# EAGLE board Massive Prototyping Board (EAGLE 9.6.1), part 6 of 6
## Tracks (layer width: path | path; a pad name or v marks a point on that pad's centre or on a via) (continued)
N$2069  (via drill 0.94) (continued)
  Bottom 2.032: v19.05,101.6 v21.59,101.6 v24.13,101.6 v26.67,101.6 v29.21,101.6
N$2070  (via drill 0.94)
  Bottom 2.032: v19.05,104.14 v21.59,104.14 v24.13,104.14 v26.67,104.14 v29.21,104.14
N$2071  (via drill 0.94)
  Bottom 2.032: v19.05,106.68 v21.59,106.68 v24.13,106.68 v26.67,106.68 v29.21,106.68
N$2072  (via drill 0.94)
  Bottom 2.032: v19.05,109.22 v21.59,109.22 v24.13,109.22 v26.67,109.22 v29.21,109.22
N$2073  (via drill 0.94)
  Bottom 2.032: v19.05,111.76 v21.59,111.76 v24.13,111.76 v26.67,111.76 v29.21,111.76
N$2074  (via drill 0.94)
  Bottom 2.032: v19.05,114.3 v21.59,114.3 v24.13,114.3 v26.67,114.3 v29.21,114.3
N$2075  (via drill 0.94)
  Bottom 2.032: v19.05,116.84 v21.59,116.84 v24.13,116.84 v26.67,116.84 v29.21,116.84
N$2076  (via drill 0.94)
  Bottom 2.032: v19.05,119.38 v21.59,119.38 v24.13,119.38 v26.67,119.38 v29.21,119.38
N$2077  (via drill 0.94)
  Bottom 2.032: v19.05,121.92 v21.59,121.92 v24.13,121.92 v26.67,121.92 v29.21,121.92
N$2078  (via drill 0.94)
  Bottom 2.032: v19.05,124.46 v21.59,124.46 v24.13,124.46 v26.67,124.46 v29.21,124.46
N$2079  (via drill 0.94)
  Bottom 2.032: v19.05,127 v21.59,127 v24.13,127 v26.67,127 v29.21,127
N$2080  (via drill 0.94)
  Bottom 2.032: v19.05,129.54 v21.59,129.54 v24.13,129.54 v26.67,129.54 v29.21,129.54
N$2081  (via drill 0.94)
  Bottom 2.032: v19.05,132.08 v21.59,132.08 v24.13,132.08 v26.67,132.08 v29.21,132.08
N$2082  (via drill 0.94)
  Bottom 2.032: v19.05,134.62 v21.59,134.62 v24.13,134.62 v26.67,134.62 v29.21,134.62
N$2083  (via drill 0.94)
  Bottom 2.032: v19.05,137.16 v21.59,137.16 v24.13,137.16 v26.67,137.16 v29.21,137.16
N$2084  (via drill 0.94)
  Bottom 2.032: v19.05,139.7 v21.59,139.7 v24.13,139.7 v26.67,139.7 v29.21,139.7
N$2085  (via drill 0.94)
  Bottom 2.032: v19.05,142.24 v21.59,142.24 v24.13,142.24 v26.67,142.24 v29.21,142.24
N$2086  (via drill 0.94)
  Bottom 2.032: v19.05,144.78 v21.59,144.78 v24.13,144.78 v26.67,144.78 v29.21,144.78
N$2087  (via drill 0.94)
  Bottom 2.032: v19.05,147.32 v21.59,147.32 v24.13,147.32 v26.67,147.32 v29.21,147.32
N$2088  (via drill 0.94)
  Bottom 2.032: v19.05,149.86 v21.59,149.86 v24.13,149.86 v26.67,149.86 v29.21,149.86
N$2089  (via drill 0.94)
  Bottom 2.032: v19.05,152.4 v21.59,152.4 v24.13,152.4 v26.67,152.4 v29.21,152.4
N$2090  (via drill 0.94)
  Bottom 2.032: v19.05,154.94 v21.59,154.94 v24.13,154.94 v26.67,154.94 v29.21,154.94
N$2091  (via drill 0.94)
  Bottom 2.032: v19.05,157.48 v21.59,157.48 v24.13,157.48 v26.67,157.48 v29.21,157.48
N$2092  (via drill 0.94)
  Bottom 2.032: v19.05,160.02 v21.59,160.02 v24.13,160.02 v26.67,160.02 v29.21,160.02
N$2093  (via drill 0.94)
  Bottom 2.032: v19.05,162.56 v21.59,162.56 v24.13,162.56 v26.67,162.56 v29.21,162.56
N$2094  (via drill 0.94)
  Bottom 2.032: v19.05,165.1 v21.59,165.1 v24.13,165.1 v26.67,165.1 v29.21,165.1
N$2095  (via drill 0.94)
  Bottom 2.032: v19.05,167.64 v21.59,167.64 v24.13,167.64 v26.67,167.64 v29.21,167.64
N$2096  (via drill 0.94)
  Bottom 2.032: v19.05,170.18 v21.59,170.18 v24.13,170.18 v26.67,170.18 v29.21,170.18
N$2097  (via drill 0.94)
  Bottom 2.032: v19.05,172.72 v21.59,172.72 v24.13,172.72 v26.67,172.72 v29.21,172.72
N$2098  (via drill 0.94)
  Bottom 2.032: v19.05,175.26 v21.59,175.26 v24.13,175.26 v26.67,175.26 v29.21,175.26
N$2099  (via drill 0.94)
  Bottom 2.032: v19.05,177.8 v21.59,177.8 v24.13,177.8 v26.67,177.8 v29.21,177.8
N$2100  (via drill 0.94)
  Bottom 2.032: v19.05,180.34 v21.59,180.34 v24.13,180.34 v26.67,180.34 v29.21,180.34
N$2101  (via drill 0.94)
  Bottom 2.032: v19.05,182.88 v21.59,182.88 v24.13,182.88 v26.67,182.88 v29.21,182.88
N$2102  (via drill 0.94)
  Bottom 2.032: v19.05,185.42 v21.59,185.42 v24.13,185.42 v26.67,185.42 v29.21,185.42
N$2103  (via drill 0.94)
  Bottom 2.032: v19.05,187.96 v21.59,187.96 v24.13,187.96 v26.67,187.96 v29.21,187.96
N$2104  (via drill 0.94)
  Bottom 2.032: v19.05,190.5 v21.59,190.5 v24.13,190.5 v26.67,190.5 v29.21,190.5
N$2105  (via drill 0.94)
  Bottom 2.032: v19.05,193.04 v21.59,193.04 v24.13,193.04 v26.67,193.04 v29.21,193.04
N$2106  (via drill 0.94)
  Bottom 2.032: v19.05,195.58 v21.59,195.58 v24.13,195.58 v26.67,195.58 v29.21,195.58
N$2107  (via drill 0.94)
  Bottom 2.032: v19.05,198.12 v21.59,198.12 v24.13,198.12 v26.67,198.12 v29.21,198.12
N$2108  (via drill 0.94)
  Bottom 2.032: v19.05,200.66 v21.59,200.66 v24.13,200.66 v26.67,200.66 v29.21,200.66
N$2109  (via drill 0.94)
  Bottom 2.032: v19.05,203.2 v21.59,203.2 v24.13,203.2 v26.67,203.2 v29.21,203.2
N$2110  (via drill 0.94)
  Bottom 2.032: v19.05,205.74 v21.59,205.74 v24.13,205.74 v26.67,205.74 v29.21,205.74
N$2111  (via drill 0.94)
  Bottom 2.032: v19.05,208.28 v21.59,208.28 v24.13,208.28 v26.67,208.28 v29.21,208.28
N$2112  (via drill 0.94)
  Bottom 2.032: v19.05,210.82 v21.59,210.82 v24.13,210.82 v26.67,210.82 v29.21,210.82
N$2113  (via drill 0.94)
  Bottom 2.032: v19.05,213.36 v21.59,213.36 v24.13,213.36 v26.67,213.36 v29.21,213.36
N$2114  (via drill 0.94)
  Bottom 2.032: v19.05,215.9 v21.59,215.9 v24.13,215.9 v26.67,215.9 v29.21,215.9
N$2115  (via drill 0.94)
  Bottom 2.032: v19.05,218.44 v21.59,218.44 v24.13,218.44 v26.67,218.44 v29.21,218.44
N$2116  (via drill 0.94)
  Bottom 2.032: v19.05,220.98 v21.59,220.98 v24.13,220.98 v26.67,220.98 v29.21,220.98
N$2117  (via drill 0.94)
  Bottom 2.032: v19.05,223.52 v21.59,223.52 v24.13,223.52 v26.67,223.52 v29.21,223.52
N$2118  (via drill 0.94)
  Bottom 2.032: v19.05,226.06 v21.59,226.06 v24.13,226.06 v26.67,226.06 v29.21,226.06
N$2119  (via drill 0.94)
  Bottom 2.032: v19.05,228.6 v21.59,228.6 v24.13,228.6 v26.67,228.6 v29.21,228.6
N$2120  (via drill 0.94)
  Bottom 2.032: v19.05,231.14 v21.59,231.14 v24.13,231.14 v26.67,231.14 v29.21,231.14
N$2121  (via drill 0.94)
  Bottom 2.032: v19.05,233.68 v21.59,233.68 v24.13,233.68 v26.67,233.68 v29.21,233.68
N$2122  (via drill 0.94)
  Bottom 2.032: v19.05,236.22 v21.59,236.22 v24.13,236.22 v26.67,236.22 v29.21,236.22
N$2123  (via drill 0.94)
  Bottom 2.032: v19.05,238.76 v21.59,238.76 v24.13,238.76 v26.67,238.76 v29.21,238.76
N$2124  (via drill 0.94)
  Bottom 2.032: v19.05,241.3 v21.59,241.3 v24.13,241.3 v26.67,241.3 v29.21,241.3
N$2125  (via drill 0.94)
  Bottom 2.032: v19.05,243.84 v21.59,243.84 v24.13,243.84 v26.67,243.84 v29.21,243.84
N$2126  (via drill 0.94)
  Bottom 2.032: v19.05,246.38 v21.59,246.38 v24.13,246.38 v26.67,246.38 v29.21,246.38
N$2127  (via drill 0.94)
  Bottom 2.032: v19.05,248.92 v21.59,248.92 v24.13,248.92 v26.67,248.92 v29.21,248.92
N$2128  (via drill 0.94)
  Bottom 2.032: v19.05,251.46 v21.59,251.46 v24.13,251.46 v26.67,251.46 v29.21,251.46
N$2129  (via drill 0.94)
  Bottom 2.032: v19.05,254 v21.59,254 v24.13,254 v26.67,254 v29.21,254
N$2130  (via drill 0.94)
  Bottom 2.032: v19.05,256.54 v21.59,256.54 v24.13,256.54 v26.67,256.54 v29.21,256.54
N$2131  (via drill 0.94)
  Bottom 2.032: v19.05,259.08 v21.59,259.08 v24.13,259.08 v26.67,259.08 v29.21,259.08
N$2132  (via drill 0.94)
  Bottom 2.032: v19.05,261.62 v21.59,261.62 v24.13,261.62 v26.67,261.62 v29.21,261.62
N$2133  (via drill 0.94)
  Bottom 2.032: v19.05,264.16 v21.59,264.16 v24.13,264.16 v26.67,264.16 v29.21,264.16
N$2134  (via drill 0.94)
  Bottom 2.032: v19.05,266.7 v21.59,266.7 v24.13,266.7 v26.67,266.7 v29.21,266.7
N$2135  (via drill 0.94)
  Bottom 2.032: v19.05,269.24 v21.59,269.24 v24.13,269.24 v26.67,269.24 v29.21,269.24
N$2136  (via drill 0.94)
  Bottom 2.032: v19.05,271.78 v21.59,271.78 v24.13,271.78 v26.67,271.78 v29.21,271.78
N$2137  (via drill 0.94)
  Bottom 2.032: v19.05,274.32 v21.59,274.32 v24.13,274.32 v26.67,274.32 v29.21,274.32
N$2138  (via drill 0.94)
  Bottom 2.032: v19.05,276.86 v21.59,276.86 v24.13,276.86 v26.67,276.86 v29.21,276.86
N$2139  (via drill 0.94)
  Bottom 2.032: v19.05,10.16 v21.59,10.16 v24.13,10.16 v26.67,10.16 v29.21,10.16
N$2140  (via drill 0.94)
  Bottom 2.032: v19.05,279.4 v21.59,279.4 v24.13,279.4 v26.67,279.4 v29.21,279.4
N$2141  (via drill 0.94)
  other vias: 11.44,111.12
N$2142  (via drill 0.94)
  other vias: 11.44,115.08
N$2143  (via drill 0.94)
  other vias: 11.44,119.04
N$2144  (via drill 0.94)
  other vias: 11.44,123
N$2145  (via drill 0.94)
  other vias: 11.44,126.96
N$2146  (via drill 0.94)
  other vias: 11.44,130.92
N$2147  (via drill 0.94)
  other vias: 11.44,134.88
N$2148  (via drill 0.94)
  other vias: 11.44,138.84
N$2149  (via drill 0.94)
  other vias: 11.44,142.8
N$2150  (via drill 0.94)
  other vias: 11.44,146.76
N$2151  (via drill 0.94)
  other vias: 11.44,150.72
N$2152  (via drill 0.94)
  other vias: 11.44,154.68
N$2153  (via drill 0.94)
  other vias: 11.44,158.64
N$2154  (via drill 0.94)
  other vias: 11.44,162.6
N$2155  (via drill 0.94)
  other vias: 11.44,166.56
N$2156  (via drill 0.94)
  other vias: 11.44,170.52
N$2157  (via drill 0.94)
  other vias: 11.44,174.48
N$2158  (via drill 0.94)
  other vias: 11.44,178.44
N$2159  (via drill 0.94)
  other vias: 13.98,111.12
N$2160  (via drill 0.94)
  other vias: 13.98,115.08
N$2161  (via drill 0.94)
  other vias: 13.98,119.04
N$2162  (via drill 0.94)
  other vias: 13.98,123
N$2163  (via drill 0.94)
  other vias: 13.98,126.96
N$2164  (via drill 0.94)
  other vias: 13.98,130.92
N$2165  (via drill 0.94)
  other vias: 13.98,134.88
N$2166  (via drill 0.94)
  other vias: 13.98,138.84
N$2167  (via drill 0.94)
  other vias: 13.98,142.8
N$2168  (via drill 0.94)
  other vias: 13.98,146.76
N$2169  (via drill 0.94)
  other vias: 13.98,150.72
N$2170  (via drill 0.94)
  other vias: 13.98,154.68
N$2171  (via drill 0.94)
  other vias: 13.98,158.64
N$2172  (via drill 0.94)
  other vias: 13.98,162.6
N$2173  (via drill 0.94)
  other vias: 13.98,166.56
N$2174  (via drill 0.94)
  other vias: 13.98,170.52
N$2175  (via drill 0.94)
  other vias: 13.98,174.48
N$2176  (via drill 0.94)
  other vias: 13.98,178.44
N$2177  (via drill 0.94)
  other vias: 326.4,111.12
N$2178  (via drill 0.94)
  other vias: 326.4,115.08
N$2179  (via drill 0.94)
  other vias: 326.4,119.04
N$2180  (via drill 0.94)
  other vias: 326.4,123
N$2181  (via drill 0.94)
  other vias: 326.4,126.96
N$2182  (via drill 0.94)
  other vias: 326.4,130.92
N$2183  (via drill 0.94)
  other vias: 326.4,134.88
N$2184  (via drill 0.94)
  other vias: 326.4,138.84
N$2185  (via drill 0.94)
  other vias: 326.4,142.8
N$2186  (via drill 0.94)
  other vias: 326.4,146.76
N$2187  (via drill 0.94)
  other vias: 326.4,150.72
N$2188  (via drill 0.94)
  other vias: 326.4,154.68
N$2189  (via drill 0.94)
  other vias: 326.4,158.64
N$2190  (via drill 0.94)
  other vias: 326.4,162.6
N$2191  (via drill 0.94)
  other vias: 326.4,166.56
N$2192  (via drill 0.94)
  other vias: 326.4,170.52
N$2193  (via drill 0.94)
  other vias: 326.4,174.48
N$2194  (via drill 0.94)
  other vias: 326.4,178.44
N$2195  (via drill 0.94)
  other vias: 328.94,111.12
N$2196  (via drill 0.94)
  other vias: 328.94,115.08
N$2197  (via drill 0.94)
  other vias: 328.94,119.04
N$2198  (via drill 0.94)
  other vias: 328.94,123
N$2199  (via drill 0.94)
  other vias: 328.94,126.96
N$2200  (via drill 0.94)
  other vias: 328.94,130.92
N$2201  (via drill 0.94)
  other vias: 328.94,134.88
N$2202  (via drill 0.94)
  other vias: 328.94,138.84
N$2203  (via drill 0.94)
  other vias: 328.94,142.8
N$2204  (via drill 0.94)
  other vias: 328.94,146.76
N$2205  (via drill 0.94)
  other vias: 328.94,150.72
N$2206  (via drill 0.94)
  other vias: 328.94,154.68
N$2207  (via drill 0.94)
  other vias: 328.94,158.64
N$2208  (via drill 0.94)
  other vias: 328.94,162.6
N$2209  (via drill 0.94)
  other vias: 328.94,166.56
N$2210  (via drill 0.94)
  other vias: 328.94,170.52
N$2211  (via drill 0.94)
  other vias: 328.94,174.48
N$2212  (via drill 0.94)
  other vias: 328.94,178.44
P1
  Bottom 2.032: 6.1,138.84 13.97,138.84
P2
  Bottom 2.032: 326.14,138.84 335.28,138.84
R1
  Bottom 2.032: 6.1,134.87 13.97,134.87
R2
  Bottom 2.032: 326.14,134.87 335.28,134.87
S1
  Bottom 2.032: 6.1,130.91 13.97,130.91
S2
  Bottom 2.032: 326.14,130.91 335.28,130.91
T1
  Bottom 2.032: 6.1,126.95 13.97,126.95
T2
  Bottom 2.032: 326.14,126.95 335.28,126.95
U1
  Bottom 2.032: 6.1,122.99 13.97,122.99
U2
  Bottom 2.032: 326.14,122.99 335.28,122.99
V1
  Bottom 2.032: 6.1,119.02 13.97,119.02
V2
  Bottom 2.032: 326.14,119.02 335.28,119.02
VCC  (via drill 0.94)
  Bottom 2.032: 64.77,285.75 64.77,10.16 | 95.25,285.75 95.25,10.16 | 125.73,285.75 125.73,10.16 | 156.21,285.75 156.21,10.16 | 186.69,285.75 186.69,10.16 | 217.17,285.75 217.17,10.16 | 247.65,285.75 247.65,10.16 | 278.13,285.75 278.13,10.16 | 308.61,285.75 308.61,10.16 | 34.29,285.75 v34.29,279.4 v34.29,276.86 v34.29,274.32 v34.29,271.78 v34.29,269.24 v34.29,266.7 v34.29,264.16 v34.29,261.62 v34.29,259.08 v34.29,256.54 v34.29,254 v34.29,251.46 v34.29,248.92 v34.29,246.38 v34.29,243.84 v34.29,241.3 v34.29,238.76 v34.29,236.22 v34.29,233.68 v34.29,231.14 v34.29,228.6 v34.29,226.06 v34.29,223.52 v34.29,220.98 v34.29,218.44 v34.29,215.9 v34.29,213.36 v34.29,210.82 v34.29,208.28 v34.29,205.74 v34.29,203.2 v34.29,200.66 v34.29,198.12 v34.29,195.58 v34.29,193.04 v34.29,190.5 v34.29,187.96 v34.29,185.42 v34.29,182.88 v34.29,180.34 v34.29,177.8 v34.29,175.26 v34.29,172.72 v34.29,170.18 v34.29,167.64 v34.29,165.1 v34.29,162.56 v34.29,160.02 v34.29,157.48 v34.29,154.94 v34.29,152.4 v34.29,149.86 v34.29,147.32 v34.29,144.78 v34.29,142.24 v34.29,139.7 v34.29,137.16 v34.29,134.62 v34.29,132.08 v34.29,129.54 v34.29,127 v34.29,124.46 v34.29,121.92 v34.29,119.38 v34.29,116.84 v34.29,114.3 v34.29,111.76 v34.29,109.22 v34.29,106.68 v34.29,104.14 v34.29,101.6 v34.29,99.06 v34.29,96.52 v34.29,93.98 v34.29,91.44 v34.29,88.9 v34.29,86.36 v34.29,83.82 v34.29,81.28 v34.29,78.74 v34.29,76.2 v34.29,73.66 v34.29,71.12 v34.29,68.58 v34.29,66.04 v34.29,63.5 v34.29,60.96 v34.29,58.42 v34.29,55.88 v34.29,53.34 v34.29,50.8 v34.29,48.26 v34.29,45.72 v34.29,43.18 v34.29,40.64 v34.29,38.1 v34.29,35.56 v34.29,33.02 v34.29,30.48 v34.29,27.94 v34.29,25.4 v34.29,22.86 v34.29,20.32 v34.29,17.78 v34.29,15.24 v34.29,12.7 v34.29,10.16
  Bottom 2.54: P1.A 4.83,184.15 P1.B | P2.1 335.53,184.15 P2.2
  Bottom 5.08: 4.83,184.15 8.89,184.15 13.97,189.23 13.97,280.67 19.05,285.75 34.29,285.75 64.77,285.75 95.25,285.75 125.73,285.75 156.21,285.75 186.69,285.75 217.17,285.75 247.65,285.75 278.13,285.75 308.61,285.75 321.31,285.75 326.39,280.67 326.39,189.23 331.47,184.15 335.53,184.15
VCC1  (via drill 0.94)  (106 unrouted)
  other vias: 64.77,10.16 64.77,12.7 64.77,15.24 64.77,17.78 64.77,20.32 64.77,22.86 64.77,25.4 64.77,27.94 64.77,30.48 64.77,33.02 64.77,35.56 64.77,38.1 64.77,40.64 64.77,43.18 64.77,45.72 64.77,48.26 64.77,50.8 64.77,53.34 64.77,55.88 64.77,58.42 64.77,63.5 64.77,60.96 64.77,66.04 64.77,68.58 64.77,71.12 64.77,73.66 64.77,76.2 64.77,78.74 64.77,83.82 64.77,81.28 64.77,86.36 64.77,88.9 64.77,91.44 64.77,93.98 64.77,96.52 64.77,99.06 64.77,101.6 64.77,104.14 64.77,106.68 64.77,109.22 64.77,111.76 64.77,114.3 64.77,116.84 64.77,119.38 64.77,121.92 64.77,124.46 64.77,127 64.77,129.54 64.77,132.08 64.77,134.62 64.77,137.16 64.77,139.7 64.77,142.24 64.77,144.78 64.77,147.32 64.77,149.86 64.77,152.4 64.77,154.94 64.77,157.48 64.77,160.02 64.77,162.56 64.77,165.1 64.77,167.64 64.77,170.18 64.77,172.72 64.77,175.26 64.77,177.8 64.77,180.34 64.77,185.42 64.77,182.88 64.77,187.96 64.77,190.5 64.77,193.04 64.77,195.58 64.77,198.12 64.77,200.66 64.77,203.2 64.77,205.74 64.77,208.28 64.77,210.82 64.77,213.36 64.77,215.9 64.77,218.44 64.77,220.98 64.77,223.52 64.77,226.06 64.77,228.6 64.77,231.14 64.77,233.68 64.77,236.22 64.77,238.76 64.77,241.3 64.77,243.84 64.77,246.38 64.77,248.92 64.77,251.46 64.77,254 64.77,256.54 64.77,259.08 64.77,261.62 64.77,264.16 64.77,266.7 64.77,269.24 64.77,271.78 64.77,274.32 64.77,276.86 64.77,279.4
VCC2  (via drill 0.94)  (106 unrouted)
  other vias: 95.25,10.16 95.25,12.7 95.25,15.24 95.25,17.78 95.25,20.32 95.25,22.86 95.25,25.4 95.25,27.94 95.25,30.48 95.25,33.02 95.25,35.56 95.25,38.1 95.25,40.64 95.25,43.18 95.25,45.72 95.25,48.26 95.25,50.8 95.25,53.34 95.25,55.88 95.25,58.42 95.25,63.5 95.25,60.96 95.25,66.04 95.25,68.58 95.25,71.12 95.25,73.66 95.25,76.2 95.25,78.74 95.25,83.82 95.25,81.28 95.25,86.36 95.25,88.9 95.25,91.44 95.25,93.98 95.25,96.52 95.25,99.06 95.25,101.6 95.25,104.14 95.25,106.68 95.25,109.22 95.25,111.76 95.25,114.3 95.25,116.84 95.25,119.38 95.25,121.92 95.25,124.46 95.25,127 95.25,129.54 95.25,132.08 95.25,134.62 95.25,137.16 95.25,139.7 95.25,142.24 95.25,144.78 95.25,147.32 95.25,149.86 95.25,152.4 95.25,154.94 95.25,157.48 95.25,160.02 95.25,162.56 95.25,165.1 95.25,167.64 95.25,170.18 95.25,172.72 95.25,175.26 95.25,177.8 95.25,180.34 95.25,185.42 95.25,182.88 95.25,187.96 95.25,190.5 95.25,193.04 95.25,195.58 95.25,198.12 95.25,200.66 95.25,203.2 95.25,205.74 95.25,208.28 95.25,210.82 95.25,213.36 95.25,215.9 95.25,218.44 95.25,220.98 95.25,223.52 95.25,226.06 95.25,228.6 95.25,231.14 95.25,233.68 95.25,236.22 95.25,238.76 95.25,241.3 95.25,243.84 95.25,246.38 95.25,248.92 95.25,251.46 95.25,254 95.25,256.54 95.25,259.08 95.25,261.62 95.25,264.16 95.25,266.7 95.25,269.24 95.25,271.78 95.25,274.32 95.25,276.86 95.25,279.4
VCC3  (via drill 0.94)  (106 unrouted)
  other vias: 125.73,10.16 125.73,12.7 125.73,15.24 125.73,17.78 125.73,20.32 125.73,22.86 125.73,25.4 125.73,27.94 125.73,30.48 125.73,33.02 125.73,35.56 125.73,38.1 125.73,40.64 125.73,43.18 125.73,45.72 125.73,48.26 125.73,50.8 125.73,53.34 125.73,55.88 125.73,58.42 125.73,63.5 125.73,60.96 125.73,66.04 125.73,68.58 125.73,71.12 125.73,73.66 125.73,76.2 125.73,78.74 125.73,83.82 125.73,81.28 125.73,86.36 125.73,88.9 125.73,91.44 125.73,93.98 125.73,96.52 125.73,99.06 125.73,101.6 125.73,104.14 125.73,106.68 125.73,109.22 125.73,111.76 125.73,114.3 125.73,116.84 125.73,119.38 125.73,121.92 125.73,124.46 125.73,127 125.73,129.54 125.73,132.08 125.73,134.62 125.73,137.16 125.73,139.7 125.73,142.24 125.73,144.78 125.73,147.32 125.73,149.86 125.73,152.4 125.73,154.94 125.73,157.48 125.73,160.02 125.73,162.56 125.73,165.1 125.73,167.64 125.73,170.18 125.73,172.72 125.73,175.26 125.73,177.8 125.73,180.34 125.73,185.42 125.73,182.88 125.73,187.96 125.73,190.5 125.73,193.04 125.73,195.58 125.73,198.12 125.73,200.66 125.73,203.2 125.73,205.74 125.73,208.28 125.73,210.82 125.73,213.36 125.73,215.9 125.73,218.44 125.73,220.98 125.73,223.52 125.73,226.06 125.73,228.6 125.73,231.14 125.73,233.68 125.73,236.22 125.73,238.76 125.73,241.3 125.73,243.84 125.73,246.38 125.73,248.92 125.73,251.46 125.73,254 125.73,256.54 125.73,259.08 125.73,261.62 125.73,264.16 125.73,266.7 125.73,269.24 125.73,271.78 125.73,274.32 125.73,276.86 125.73,279.4
VCC4  (via drill 0.94)  (106 unrouted)
  other vias: 156.21,10.16 156.21,12.7 156.21,15.24 156.21,17.78 156.21,20.32 156.21,22.86 156.21,25.4 156.21,27.94 156.21,30.48 156.21,33.02 156.21,35.56 156.21,38.1 156.21,40.64 156.21,43.18 156.21,45.72 156.21,48.26 156.21,50.8 156.21,53.34 156.21,55.88 156.21,58.42 156.21,63.5 156.21,60.96 156.21,66.04 156.21,68.58 156.21,71.12 156.21,73.66 156.21,76.2 156.21,78.74 156.21,83.82 156.21,81.28 156.21,86.36 156.21,88.9 156.21,91.44 156.21,93.98 156.21,96.52 156.21,99.06 156.21,101.6 156.21,104.14 156.21,106.68 156.21,109.22 156.21,111.76 156.21,114.3 156.21,116.84 156.21,119.38 156.21,121.92 156.21,124.46 156.21,127 156.21,129.54 156.21,132.08 156.21,134.62 156.21,137.16 156.21,139.7 156.21,142.24 156.21,144.78 156.21,147.32 156.21,149.86 156.21,152.4 156.21,154.94 156.21,157.48 156.21,160.02 156.21,162.56 156.21,165.1 156.21,167.64 156.21,170.18 156.21,172.72 156.21,175.26 156.21,177.8 156.21,180.34 156.21,185.42 156.21,182.88 156.21,187.96 156.21,190.5 156.21,193.04 156.21,195.58 156.21,198.12 156.21,200.66 156.21,203.2 156.21,205.74 156.21,208.28 156.21,210.82 156.21,213.36 156.21,215.9 156.21,218.44 156.21,220.98 156.21,223.52 156.21,226.06 156.21,228.6 156.21,231.14 156.21,233.68 156.21,236.22 156.21,238.76 156.21,241.3 156.21,243.84 156.21,246.38 156.21,248.92 156.21,251.46 156.21,254 156.21,256.54 156.21,259.08 156.21,261.62 156.21,264.16 156.21,266.7 156.21,269.24 156.21,271.78 156.21,274.32 156.21,276.86 156.21,279.4
VCC5  (via drill 0.94)  (106 unrouted)
  other vias: 186.69,10.16 186.69,12.7 186.69,15.24 186.69,17.78 186.69,20.32 186.69,22.86 186.69,25.4 186.69,27.94 186.69,30.48 186.69,33.02 186.69,35.56 186.69,38.1 186.69,40.64 186.69,43.18 186.69,45.72 186.69,48.26 186.69,50.8 186.69,53.34 186.69,55.88 186.69,58.42 186.69,63.5 186.69,60.96 186.69,66.04 186.69,68.58 186.69,71.12 186.69,73.66 186.69,76.2 186.69,78.74 186.69,83.82 186.69,81.28 186.69,86.36 186.69,88.9 186.69,91.44 186.69,93.98 186.69,96.52 186.69,99.06 186.69,101.6 186.69,104.14 186.69,106.68 186.69,109.22 186.69,111.76 186.69,114.3 186.69,116.84 186.69,119.38 186.69,121.92 186.69,124.46 186.69,127 186.69,129.54 186.69,132.08 186.69,134.62 186.69,137.16 186.69,139.7 186.69,142.24 186.69,144.78 186.69,147.32 186.69,149.86 186.69,152.4 186.69,154.94 186.69,157.48 186.69,160.02 186.69,162.56 186.69,165.1 186.69,167.64 186.69,170.18 186.69,172.72 186.69,175.26 186.69,177.8 186.69,180.34 186.69,185.42 186.69,182.88 186.69,187.96 186.69,190.5 186.69,193.04 186.69,195.58 186.69,198.12 186.69,200.66 186.69,203.2 186.69,205.74 186.69,208.28 186.69,210.82 186.69,213.36 186.69,215.9 186.69,218.44 186.69,220.98 186.69,223.52 186.69,226.06 186.69,228.6 186.69,231.14 186.69,233.68 186.69,236.22 186.69,238.76 186.69,241.3 186.69,243.84 186.69,246.38 186.69,248.92 186.69,251.46 186.69,254 186.69,256.54 186.69,259.08 186.69,261.62 186.69,264.16 186.69,266.7 186.69,269.24 186.69,271.78 186.69,274.32 186.69,276.86 186.69,279.4
VCC6  (via drill 0.94)  (106 unrouted)
  other vias: 217.17,10.16 217.17,12.7 217.17,15.24 217.17,17.78 217.17,20.32 217.17,22.86 217.17,25.4 217.17,27.94 217.17,30.48 217.17,33.02 217.17,35.56 217.17,38.1 217.17,40.64 217.17,43.18 217.17,45.72 217.17,48.26 217.17,50.8 217.17,53.34 217.17,55.88 217.17,58.42 217.17,63.5 217.17,60.96 217.17,66.04 217.17,68.58 217.17,71.12 217.17,73.66 217.17,76.2 217.17,78.74 217.17,83.82 217.17,81.28 217.17,86.36 217.17,88.9 217.17,91.44 217.17,93.98 217.17,96.52 217.17,99.06 217.17,101.6 217.17,104.14 217.17,106.68 217.17,109.22 217.17,111.76 217.17,114.3 217.17,116.84 217.17,119.38 217.17,121.92 217.17,124.46 217.17,127 217.17,129.54 217.17,132.08 217.17,134.62 217.17,137.16 217.17,139.7 217.17,142.24 217.17,144.78 217.17,147.32 217.17,149.86 217.17,152.4 217.17,154.94 217.17,157.48 217.17,160.02 217.17,162.56 217.17,165.1 217.17,167.64 217.17,170.18 217.17,172.72 217.17,175.26 217.17,177.8 217.17,180.34 217.17,185.42 217.17,182.88 217.17,187.96 217.17,190.5 217.17,193.04 217.17,195.58 217.17,198.12 217.17,200.66 217.17,203.2 217.17,205.74 217.17,208.28 217.17,210.82 217.17,213.36 217.17,215.9 217.17,218.44 217.17,220.98 217.17,223.52 217.17,226.06 217.17,228.6 217.17,231.14 217.17,233.68 217.17,236.22 217.17,238.76 217.17,241.3 217.17,243.84 217.17,246.38 217.17,248.92 217.17,251.46 217.17,254 217.17,256.54 217.17,259.08 217.17,261.62 217.17,264.16 217.17,266.7 217.17,269.24 217.17,271.78 217.17,274.32 217.17,276.86 217.17,279.4
VCC7  (via drill 0.94)  (106 unrouted)
  other vias: 247.65,10.16 247.65,12.7 247.65,15.24 247.65,17.78 247.65,20.32 247.65,22.86 247.65,25.4 247.65,27.94 247.65,30.48 247.65,33.02 247.65,35.56 247.65,38.1 247.65,40.64 247.65,43.18 247.65,45.72 247.65,48.26 247.65,50.8 247.65,53.34 247.65,55.88 247.65,58.42 247.65,63.5 247.65,60.96 247.65,66.04 247.65,68.58 247.65,71.12 247.65,73.66 247.65,76.2 247.65,78.74 247.65,83.82 247.65,81.28 247.65,86.36 247.65,88.9 247.65,91.44 247.65,93.98 247.65,96.52 247.65,99.06 247.65,101.6 247.65,104.14 247.65,106.68 247.65,109.22 247.65,111.76 247.65,114.3 247.65,116.84 247.65,119.38 247.65,121.92 247.65,124.46 247.65,127 247.65,129.54 247.65,132.08 247.65,134.62 247.65,137.16 247.65,139.7 247.65,142.24 247.65,144.78 247.65,147.32 247.65,149.86 247.65,152.4 247.65,154.94 247.65,157.48 247.65,160.02 247.65,162.56 247.65,165.1 247.65,167.64 247.65,170.18 247.65,172.72 247.65,175.26 247.65,177.8 247.65,180.34 247.65,185.42 247.65,182.88 247.65,187.96 247.65,190.5 247.65,193.04 247.65,195.58 247.65,198.12 247.65,200.66 247.65,203.2 247.65,205.74 247.65,208.28 247.65,210.82 247.65,213.36 247.65,215.9 247.65,218.44 247.65,220.98 247.65,223.52 247.65,226.06 247.65,228.6 247.65,231.14 247.65,233.68 247.65,236.22 247.65,238.76 247.65,241.3 247.65,243.84 247.65,246.38 247.65,248.92 247.65,251.46 247.65,254 247.65,256.54 247.65,259.08 247.65,261.62 247.65,264.16 247.65,266.7 247.65,269.24 247.65,271.78 247.65,274.32 247.65,276.86 247.65,279.4
VCC8  (via drill 0.94)  (106 unrouted)
  other vias: 278.13,10.16 278.13,12.7 278.13,15.24 278.13,17.78 278.13,20.32 278.13,22.86 278.13,25.4 278.13,27.94 278.13,30.48 278.13,33.02 278.13,35.56 278.13,38.1 278.13,40.64 278.13,43.18 278.13,45.72 278.13,48.26 278.13,50.8 278.13,53.34 278.13,55.88 278.13,58.42 278.13,63.5 278.13,60.96 278.13,66.04 278.13,68.58 278.13,71.12 278.13,73.66 278.13,76.2 278.13,78.74 278.13,83.82 278.13,81.28 278.13,86.36 278.13,88.9 278.13,91.44 278.13,93.98 278.13,96.52 278.13,99.06 278.13,101.6 278.13,104.14 278.13,106.68 278.13,109.22 278.13,111.76 278.13,114.3 278.13,116.84 278.13,119.38 278.13,121.92 278.13,124.46 278.13,127 278.13,129.54 278.13,132.08 278.13,134.62 278.13,137.16 278.13,139.7 278.13,142.24 278.13,144.78 278.13,147.32 278.13,149.86 278.13,152.4 278.13,154.94 278.13,157.48 278.13,160.02 278.13,162.56 278.13,165.1 278.13,167.64 278.13,170.18 278.13,172.72 278.13,175.26 278.13,177.8 278.13,180.34 278.13,185.42 278.13,182.88 278.13,187.96 278.13,190.5 278.13,193.04 278.13,195.58 278.13,198.12 278.13,200.66 278.13,203.2 278.13,205.74 278.13,208.28 278.13,210.82 278.13,213.36 278.13,215.9 278.13,218.44 278.13,220.98 278.13,223.52 278.13,226.06 278.13,228.6 278.13,231.14 278.13,233.68 278.13,236.22 278.13,238.76 278.13,241.3 278.13,243.84 278.13,246.38 278.13,248.92 278.13,251.46 278.13,254 278.13,256.54 278.13,259.08 278.13,261.62 278.13,264.16 278.13,266.7 278.13,269.24 278.13,271.78 278.13,274.32 278.13,276.86 278.13,279.4
VCC9  (via drill 0.94)  (106 unrouted)
  other vias: 308.61,10.16 308.61,12.7 308.61,15.24 308.61,17.78 308.61,20.32 308.61,22.86 308.61,25.4 308.61,27.94 308.61,30.48 308.61,33.02 308.61,35.56 308.61,38.1 308.61,40.64 308.61,43.18 308.61,45.72 308.61,48.26 308.61,50.8 308.61,53.34 308.61,55.88 308.61,58.42 308.61,63.5 308.61,60.96 308.61,66.04 308.61,68.58 308.61,71.12 308.61,73.66 308.61,76.2 308.61,78.74 308.61,83.82 308.61,81.28 308.61,86.36 308.61,88.9 308.61,91.44 308.61,93.98 308.61,96.52 308.61,99.06 308.61,101.6 308.61,104.14 308.61,106.68 308.61,109.22 308.61,111.76 308.61,114.3 308.61,116.84 308.61,119.38 308.61,121.92 308.61,124.46 308.61,127 308.61,129.54 308.61,132.08 308.61,134.62 308.61,137.16 308.61,139.7 308.61,142.24 308.61,144.78 308.61,147.32 308.61,149.86 308.61,152.4 308.61,154.94 308.61,157.48 308.61,160.02 308.61,162.56 308.61,165.1 308.61,167.64 308.61,170.18 308.61,172.72 308.61,175.26 308.61,177.8 308.61,180.34 308.61,185.42 308.61,182.88 308.61,187.96 308.61,190.5 308.61,193.04 308.61,195.58 308.61,198.12 308.61,200.66 308.61,203.2 308.61,205.74 308.61,208.28 308.61,210.82 308.61,213.36 308.61,215.9 308.61,218.44 308.61,220.98 308.61,223.52 308.61,226.06 308.61,228.6 308.61,231.14 308.61,233.68 308.61,236.22 308.61,238.76 308.61,241.3 308.61,243.84 308.61,246.38 308.61,248.92 308.61,251.46 308.61,254 308.61,256.54 308.61,259.08 308.61,261.62 308.61,264.16 308.61,266.7 308.61,269.24 308.61,271.78 308.61,274.32 308.61,276.86 308.61,279.4
W1
  Bottom 2.032: 6.1,115.06 13.97,115.06
W2
  Bottom 2.032: 326.14,115.06 335.28,115.06
X1
  Bottom 2.032: 6.1,111.1 13.97,111.1
X2
  Bottom 2.032: 326.14,111.1 335.28,111.1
